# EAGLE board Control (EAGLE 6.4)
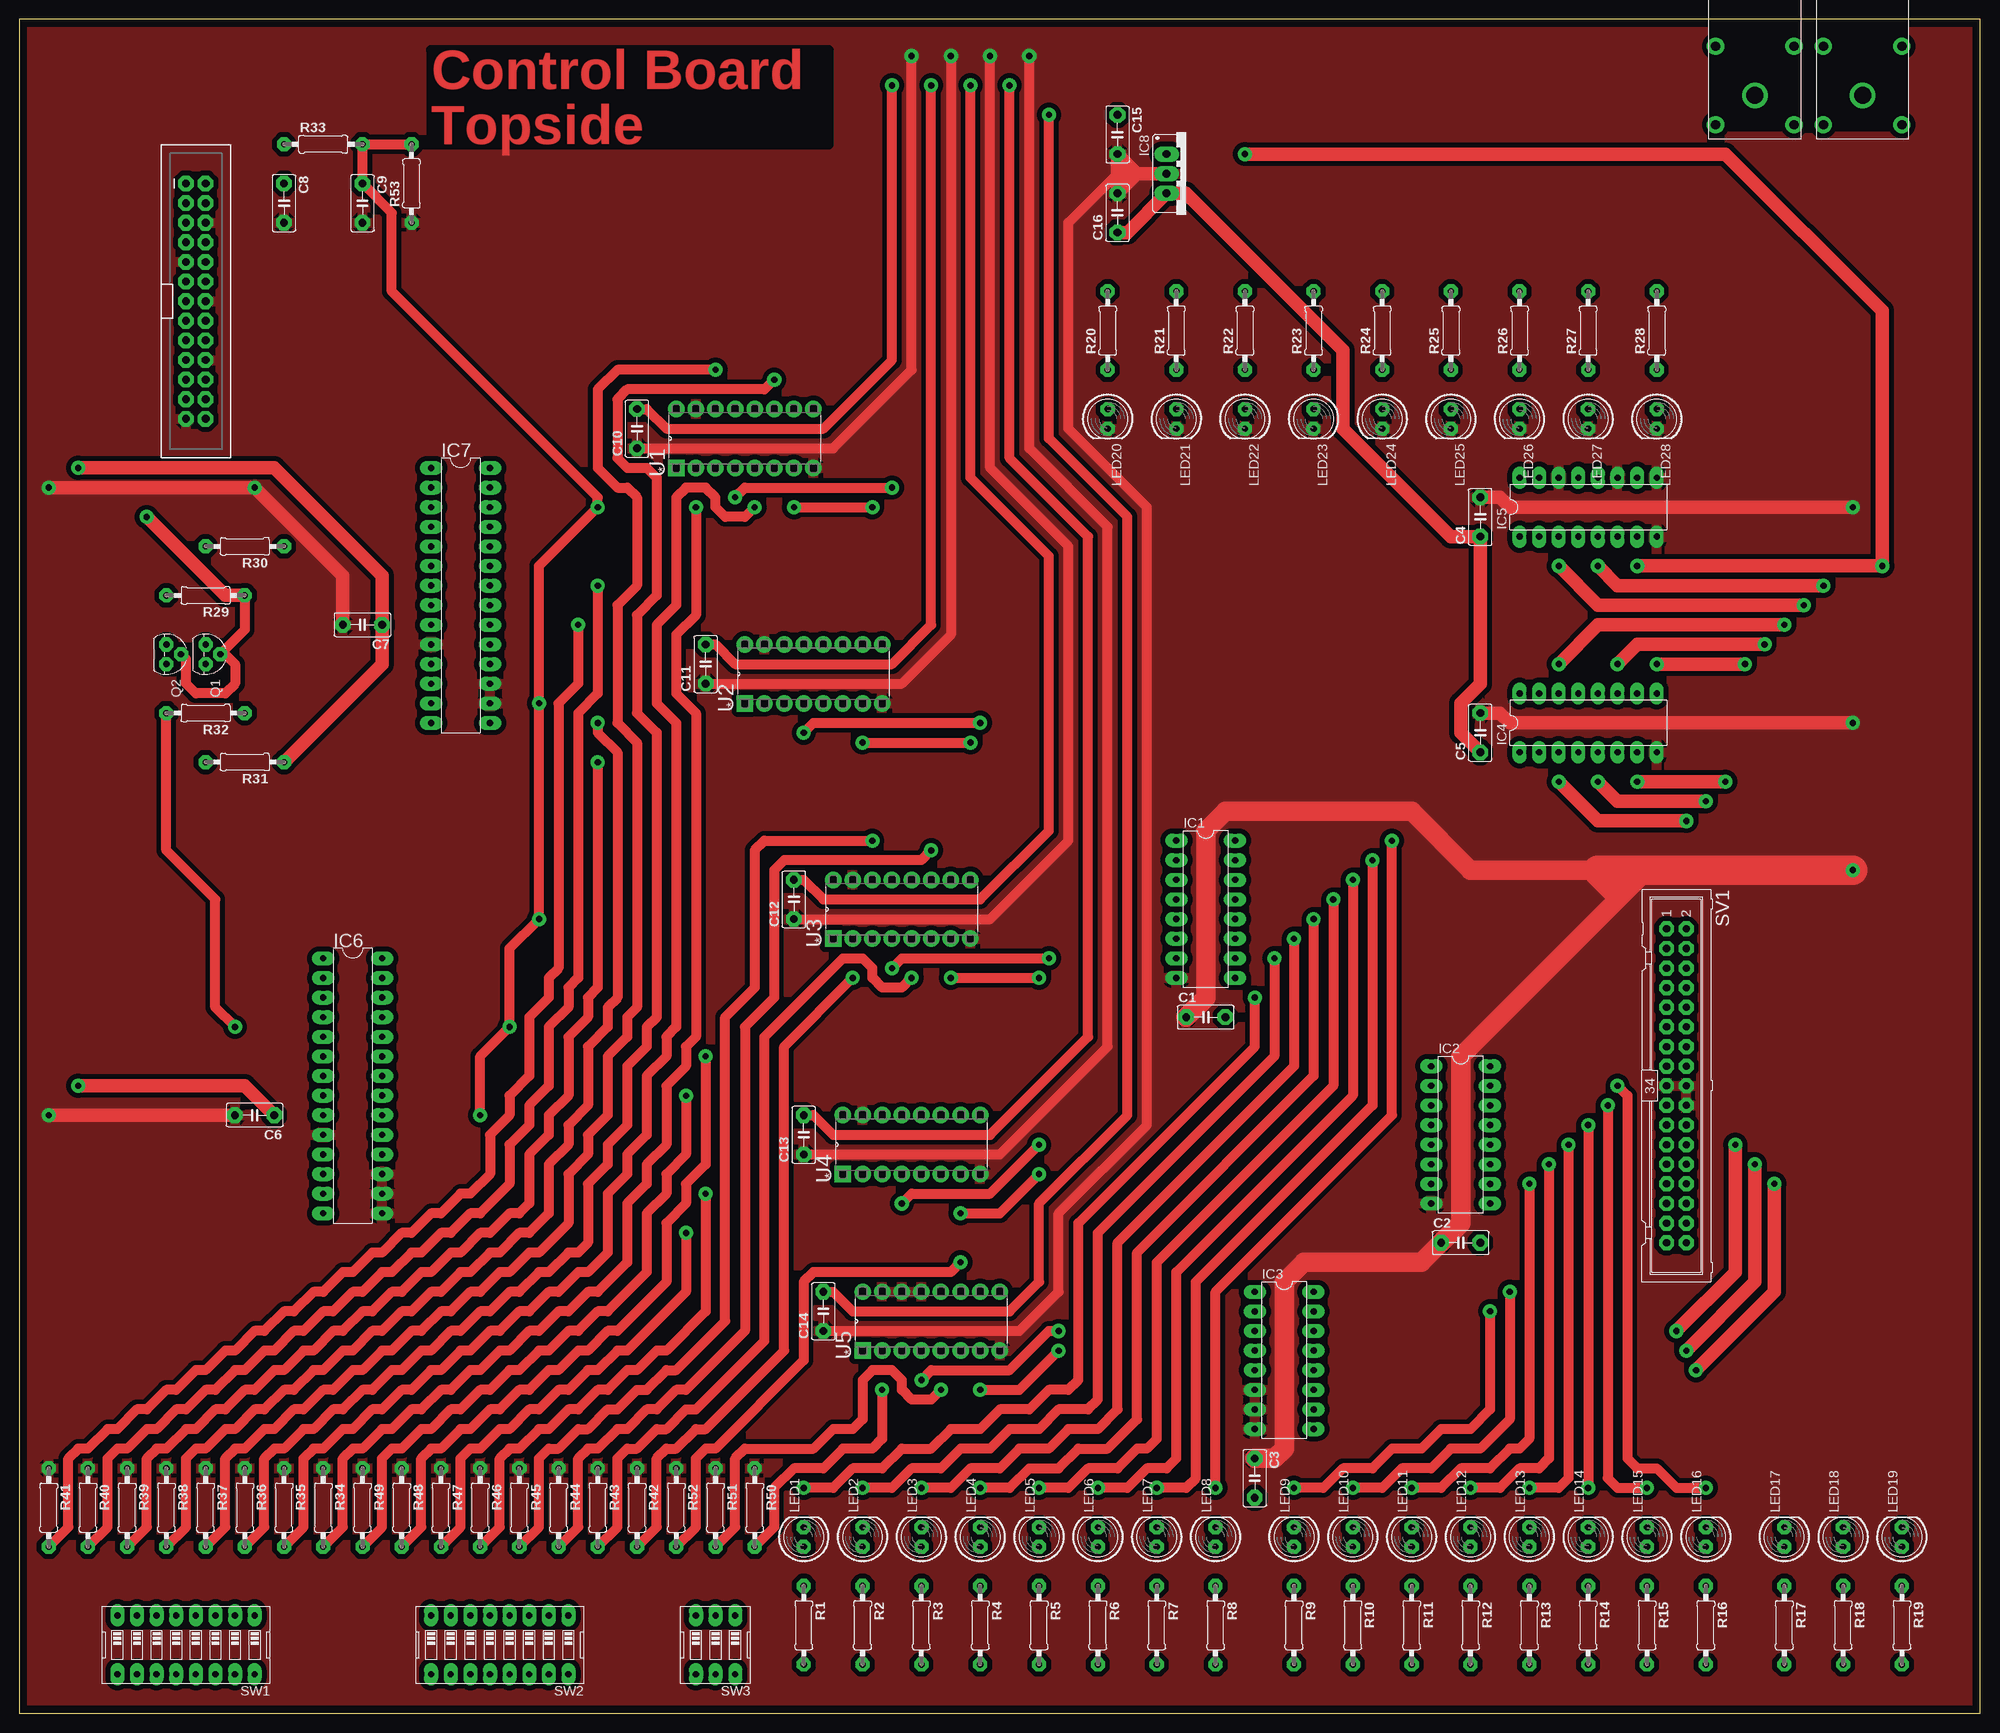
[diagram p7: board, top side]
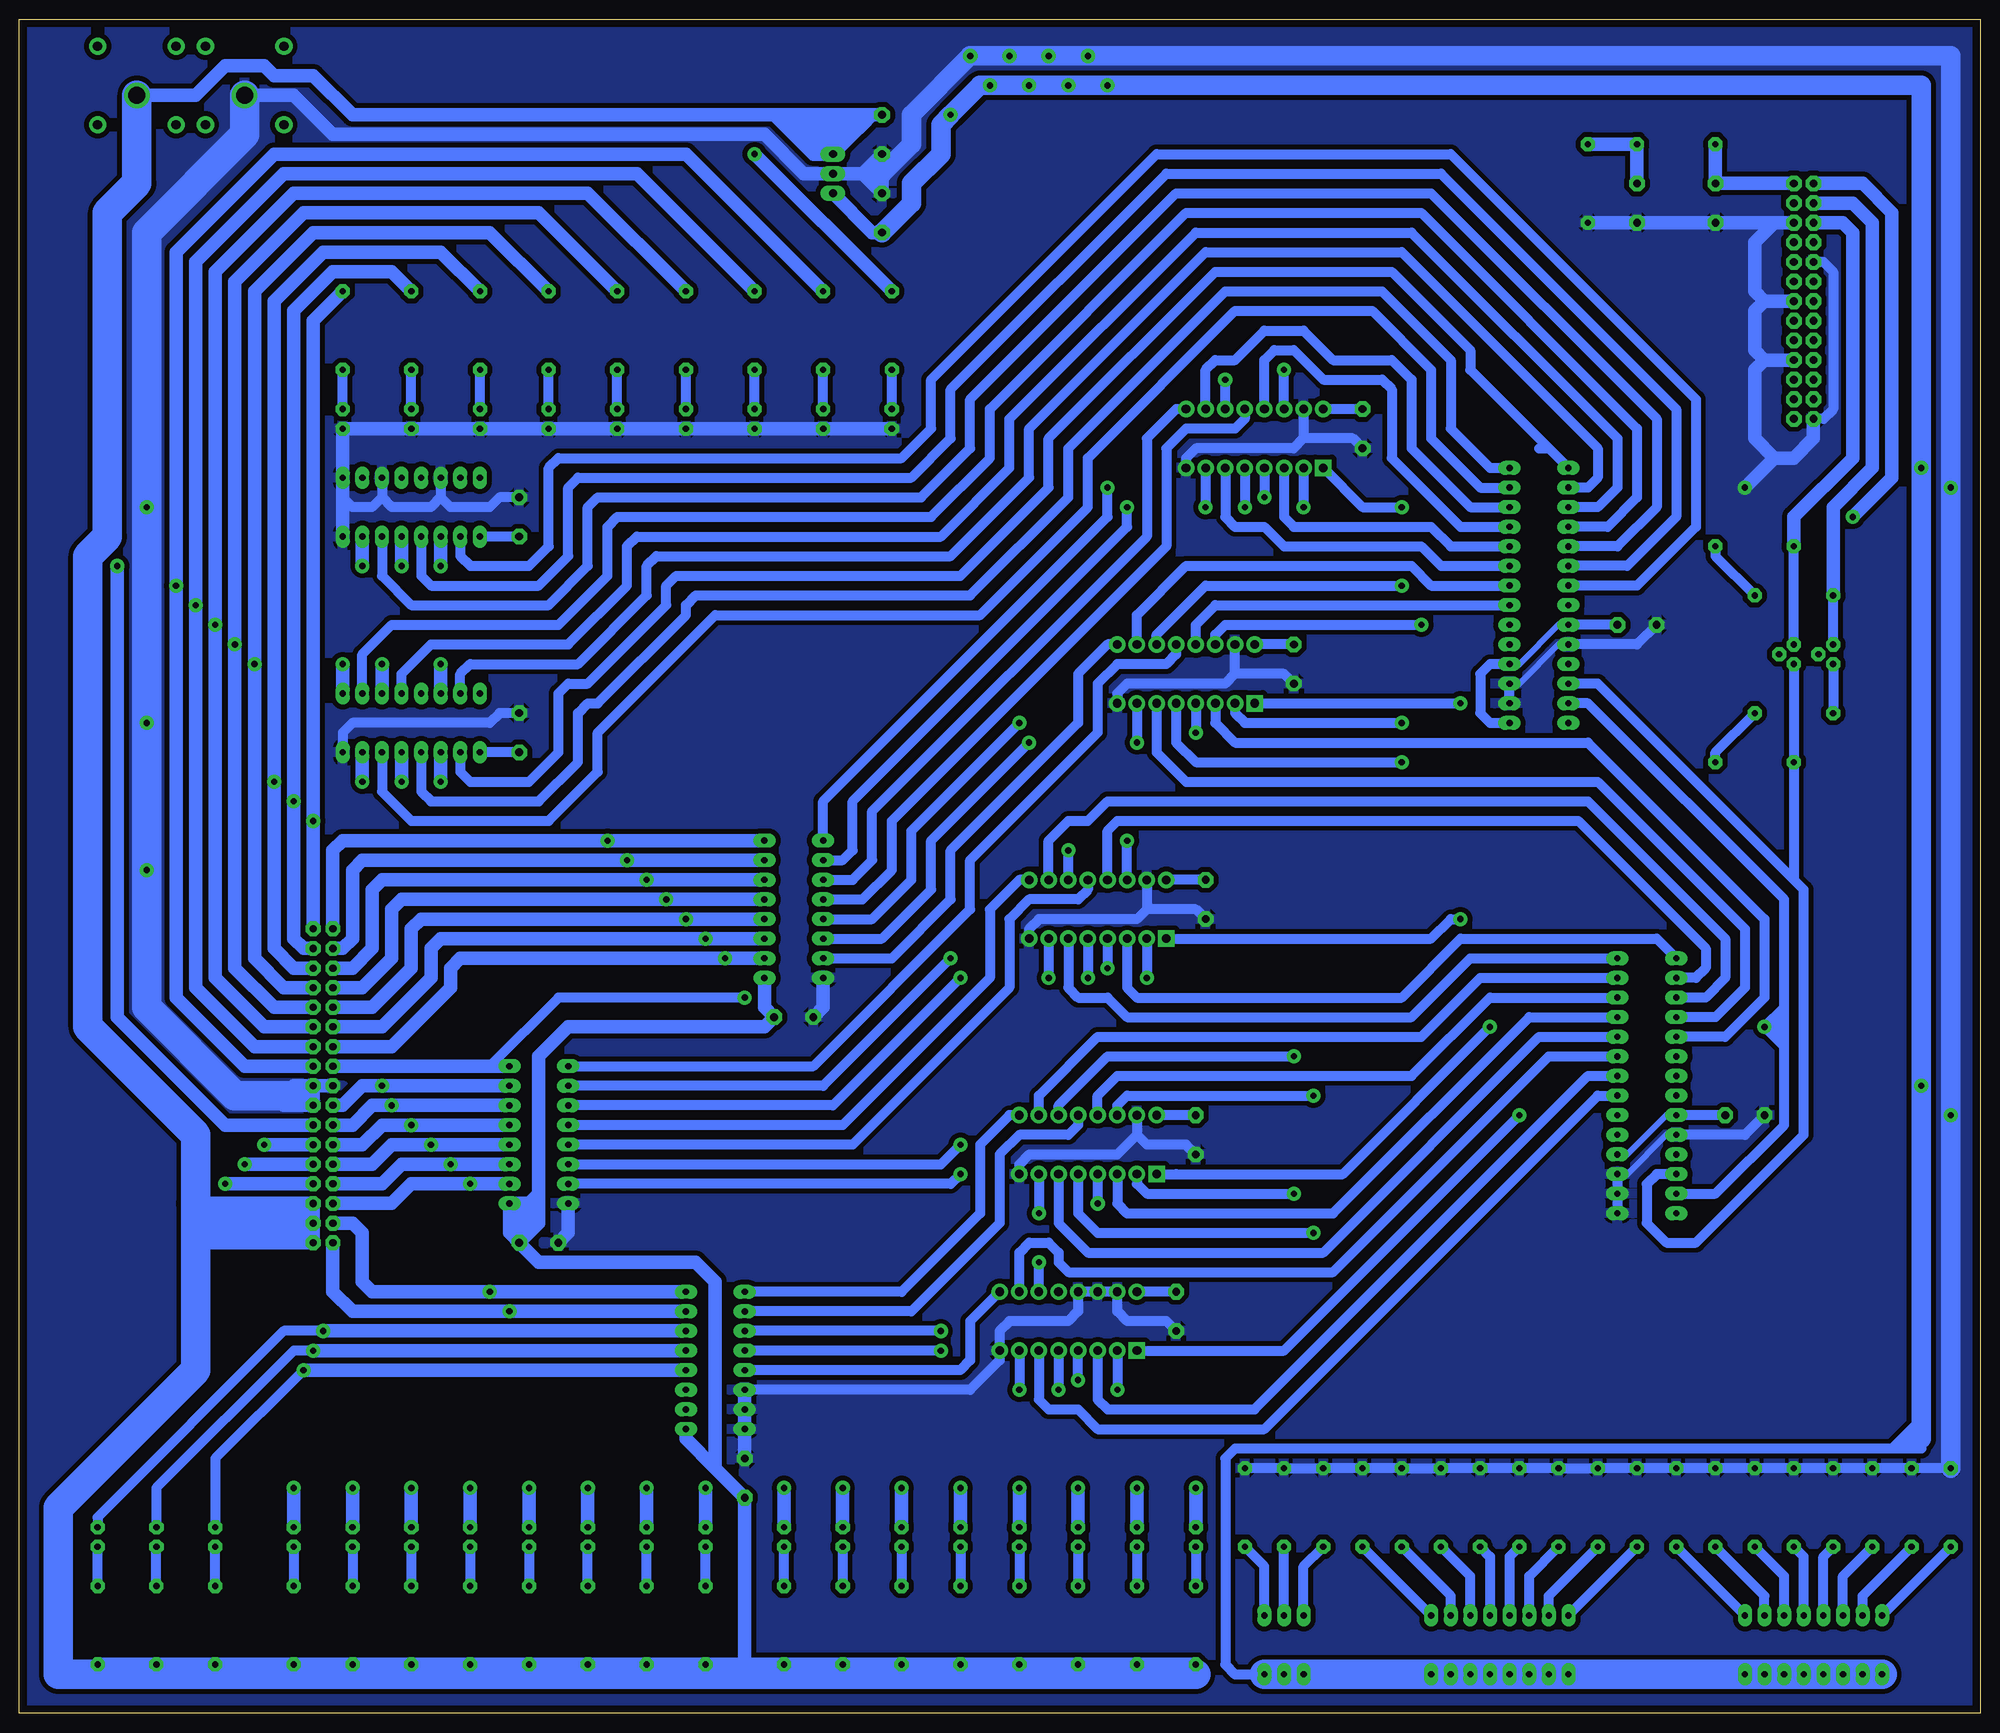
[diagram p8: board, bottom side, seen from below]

Size 253.98 x 219.38 mm. Coordinates in mm from the lower left corner, seen from the top.
Outline: 0,0 253.98,0 253.98,219.38 0,219.38 0,0
Copper layers (1*16): Top 0.035mm / dielectric 1.5mm / Bottom 0.035mm
Design rules "arm-rules-modified": minimum track width 20mil, minimum drill 24mil, track to track 25mil, track to pad 20mil, pad to pad 15mil, via to via 20mil, smd to smd 8mil, copper to edge 40mil, drill to drill 12mil, minimum pad ring 20mil, minimum via ring 20mil, stop-mask expansion 0mil, vias tented up to drill 0mil, thermal gap 15mil
Net classes: 1 12V_Power: width 0.762 mm; 2 Ground: width 0.762 mm; 3 Relay_Interconnects: width 0.762 mm

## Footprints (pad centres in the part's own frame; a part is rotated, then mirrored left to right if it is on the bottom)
C050-030-075 = drill 1 octagon: 1 -2.54,0; 2 2.54,0
DIL16 = drill 0.813 long: 1 -8.89,-3.81; 2 -6.35,-3.81; 3 -3.81,-3.81; 4 -1.27,-3.81; 5 1.27,-3.81; 6 3.81,-3.81; 7 6.35,-3.81; 8 8.89,-3.81; 9 8.89,3.81; 10 6.35,3.81; 11 3.81,3.81; 12 1.27,3.81; 13 -1.27,3.81; 14 -3.81,3.81; 15 -6.35,3.81; 16 -8.89,3.81
DIL28-3 = drill 0.813 long: 1 -16.51,-3.81; 2 -13.97,-3.81; 3 -11.43,-3.81; 4 -8.89,-3.81; 5 -6.35,-3.81; 6 -3.81,-3.81; 7 -1.27,-3.81; 8 1.27,-3.81; 9 3.81,-3.81; 10 6.35,-3.81; 11 8.89,-3.81; 12 11.43,-3.81; 13 13.97,-3.81; 14 16.51,-3.81; 15 16.51,3.81; 16 13.97,3.81; 17 11.43,3.81; 18 8.89,3.81; 19 6.35,3.81; 20 3.81,3.81; 21 1.27,3.81; 22 -1.27,3.81; 23 -3.81,3.81; 24 -6.35,3.81; 25 -8.89,3.81; 26 -11.43,3.81; 27 -13.97,3.81; 28 -16.51,3.81
78XXS = drill 1.016 long: GND 0,-2.54; IN -2.54,-2.54; OUT 2.54,-2.54
2X13-SHROUDED = drill 1.016 pad 1.88 octagon: 1 -1.27,15.24; 2 1.27,15.24; 3 -1.27,12.7; 4 1.27,12.7; 5 -1.27,10.16; 6 1.27,10.16; 7 -1.27,7.62; 8 1.27,7.62; 9 -1.27,5.08; 10 1.27,5.08; 11 -1.27,2.54; 12 1.27,2.54; 13 -1.27,0; 14 1.27,0; 15 -1.27,-2.54; 16 1.27,-2.54; 17 -1.27,-5.08; 18 1.27,-5.08; 19 -1.27,-7.62; 20 1.27,-7.62; 21 -1.27,-10.16; 22 1.27,-10.16; 23 -1.27,-12.7; 24 1.27,-12.7; 25 -1.27,-15.24; 26 1.27,-15.24
LED5MM = drill 0.813 octagon: A -1.27,0; K 1.27,0
TO-92 = drill 0.813 octagon: 1 -1.27,0; 2 0,1.905; 3 1.27,0
0207/10 = drill 0.8 octagon: 1 -5.08,0; 2 5.08,0
ML34 = drill 0.914 octagon: 1 -20.32,-1.27; 2 -20.32,1.27; 3 -17.78,-1.27; 4 -17.78,1.27; 5 -15.24,-1.27; 6 -15.24,1.27; 7 -12.7,-1.27; 8 -12.7,1.27; 9 -10.16,-1.27; 10 -10.16,1.27; 11 -7.62,-1.27; 12 -7.62,1.27; 13 -5.08,-1.27; 14 -5.08,1.27; 15 -2.54,-1.27; 16 -2.54,1.27; 17 0,-1.27; 18 0,1.27; 19 2.54,-1.27; 20 2.54,1.27; 21 5.08,-1.27; 22 5.08,1.27; 23 7.62,-1.27; 24 7.62,1.27; 25 10.16,-1.27; 26 10.16,1.27; 27 12.7,-1.27; 28 12.7,1.27; 29 15.24,-1.27; 30 15.24,1.27; 31 17.78,-1.27; 32 17.78,1.27; 33 20.32,-1.27; 34 20.32,1.27
EDG-08 = drill 0.813 long: 1 -8.89,-3.81; 2 -6.35,-3.81; 3 -3.81,-3.81; 4 -1.27,-3.81; 5 1.27,-3.81; 6 3.81,-3.81; 7 6.35,-3.81; 8 8.89,-3.81; 9 8.89,3.81; 10 6.35,3.81; 11 3.81,3.81; 12 1.27,3.81; 13 -1.27,3.81; 14 -3.81,3.81; 15 -6.35,3.81; 16 -8.89,3.81
EDG-03 = drill 0.813 long: 1 -2.54,-3.81; 2 0,-3.81; 3 2.54,-3.81; 4 2.54,3.81; 5 0,3.81; 6 -2.54,3.81
DIP254P762X508-16 = drill 1.118 square: 1 -7.62,17.78 | drill 1.118: 2 -7.62,15.24; 3 -7.62,12.7; 4 -7.62,10.16; 5 -7.62,7.62; 6 -7.62,5.08; 7 -7.62,2.54; 8 -7.62,0; 9 0,0; 10 0,2.54; 11 0,5.08; 12 0,7.62; 13 0,10.16; 14 0,12.7; 15 0,15.24; 16 0,17.78
BANPLUG = drill 2.2: 1 0,-6.36 | drill 1.2: P$1 -5.08,-10.16; P$2 5.08,-10.16; P$3 -5.08,0; P$4 5.08,0

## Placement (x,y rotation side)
C1  [C050-030-075]  153.67,90.17 0 top
C2  [C050-030-075]  186.69,60.96 0 top
C3  [C050-030-075]  160.02,30.48 270 top
C4  [C050-030-075]  189.23,154.94 90 top
C5  [C050-030-075]  189.23,127 90 top
C6  [C050-030-075]  30.48,77.47 180 top
C7  [C050-030-075]  44.45,140.97 180 top
C8  22n  [C050-030-075]  34.29,195.58 270 top
C9  22n  [C050-030-075]  44.45,195.58 270 top
C10  [C050-030-075]  80.01,166.37 90 top
C11  [C050-030-075]  88.9,135.89 90 top
C12  [C050-030-075]  100.33,105.41 90 top
C13  [C050-030-075]  101.6,74.93 90 top
C14  [C050-030-075]  104.14,52.07 90 top
C15  [C050-030-075]  142.24,204.47 270 top
C16  [C050-030-075]  142.24,194.31 90 top
IC1  ULN2003AN  [DIL16]  153.67,104.14 270 top
IC2  ULN2003AN  [DIL16]  186.69,74.93 270 top
IC3  ULN2003AN  [DIL16]  163.83,45.72 270 top
IC4  4049N  [DIL16]  203.2,128.27 0 top
IC5  4049N  [DIL16]  203.2,156.21 0 top
IC6  MCP23017SP  [DIL28-3]  43.18,81.28 270 top
IC7  MCP23017SP  [DIL28-3]  57.15,144.78 270 top
IC8  [78XXS]  151.13,199.39 270 top
JP1  RASPBERRYPI-GPIOPTH  [2X13-SHROUDED]  22.86,182.88 0 top
LED1  [LED5MM]  101.6,22.86 90 top
LED2  [LED5MM]  109.22,22.86 90 top
LED3  [LED5MM]  116.84,22.86 90 top
LED4  [LED5MM]  124.46,22.86 90 top
LED5  [LED5MM]  132.08,22.86 90 top
LED6  [LED5MM]  139.7,22.86 90 top
LED7  [LED5MM]  147.32,22.86 90 top
LED8  [LED5MM]  154.94,22.86 90 top
LED9  [LED5MM]  165.1,22.86 90 top
LED10  [LED5MM]  172.72,22.86 90 top
LED11  [LED5MM]  180.34,22.86 90 top
LED12  [LED5MM]  187.96,22.86 90 top
LED13  [LED5MM]  195.58,22.86 90 top
LED14  [LED5MM]  203.2,22.86 90 top
LED15  [LED5MM]  210.82,22.86 90 top
LED16  [LED5MM]  218.44,22.86 90 top
LED17  [LED5MM]  228.6,22.86 90 top
LED18  [LED5MM]  236.22,22.86 90 top
LED19  [LED5MM]  243.84,22.86 90 top
LED20  [LED5MM]  140.97,167.64 270 top
LED21  [LED5MM]  149.86,167.64 270 top
LED22  [LED5MM]  158.75,167.64 270 top
LED23  [LED5MM]  167.64,167.64 270 top
LED24  [LED5MM]  176.53,167.64 270 top
LED25  [LED5MM]  185.42,167.64 270 top
LED26  [LED5MM]  194.31,167.64 270 top
LED27  [LED5MM]  203.2,167.64 270 top
LED28  [LED5MM]  212.09,167.64 270 top
Q1  TN0602N3  [TO-92]  24.13,137.16 270 top
Q2  TN0602N3  [TO-92]  19.05,137.16 270 top
R1  510  [0207/10]  101.6,11.43 270 top
R2  510  [0207/10]  109.22,11.43 270 top
R3  510  [0207/10]  116.84,11.43 270 top
R4  510  [0207/10]  124.46,11.43 270 top
R5  510  [0207/10]  132.08,11.43 270 top
R6  510  [0207/10]  139.7,11.43 270 top
R7  510  [0207/10]  147.32,11.43 270 top
R8  510  [0207/10]  154.94,11.43 270 top
R9  510  [0207/10]  165.1,11.43 270 top
R10  510  [0207/10]  172.72,11.43 270 top
R11  510  [0207/10]  180.34,11.43 270 top
R12  510  [0207/10]  187.96,11.43 270 top
R13  510  [0207/10]  195.58,11.43 270 top
R14  510  [0207/10]  203.2,11.43 270 top
R15  510  [0207/10]  210.82,11.43 270 top
R16  510  [0207/10]  218.44,11.43 270 top
R17  510  [0207/10]  228.6,11.43 270 top
R18  510  [0207/10]  236.22,11.43 270 top
R19  510  [0207/10]  243.84,11.43 270 top
R20  510  [0207/10]  140.97,179.07 90 top
R21  510  [0207/10]  149.86,179.07 90 top
R22  510  [0207/10]  158.75,179.07 90 top
R23  510  [0207/10]  167.64,179.07 90 top
R24  510  [0207/10]  176.53,179.07 90 top
R25  510  [0207/10]  185.42,179.07 90 top
R26  510  [0207/10]  194.31,179.07 90 top
R27  510  [0207/10]  203.2,179.07 90 top
R28  510  [0207/10]  212.09,179.07 90 top
R29  10k  [0207/10]  24.13,144.78 180 top
R30  10k  [0207/10]  29.21,151.13 180 top
R31  10k  [0207/10]  29.21,123.19 180 top
R32  10k  [0207/10]  24.13,129.54 180 top
R33  100  [0207/10]  39.37,203.2 0 top
R34  10k  [0207/10]  39.37,26.67 270 top
R35  10k  [0207/10]  34.29,26.67 270 top
R36  10k  [0207/10]  29.21,26.67 270 top
R37  10k  [0207/10]  24.13,26.67 270 top
R38  10k  [0207/10]  19.05,26.67 270 top
R39  10k  [0207/10]  13.97,26.67 270 top
R40  10k  [0207/10]  8.89,26.67 270 top
R41  10k  [0207/10]  3.81,26.67 270 top
R42  10k  [0207/10]  80.01,26.67 270 top
R43  10k  [0207/10]  74.93,26.67 270 top
R44  10k  [0207/10]  69.85,26.67 270 top
R45  10k  [0207/10]  64.77,26.67 270 top
R46  10k  [0207/10]  59.69,26.67 270 top
R47  10k  [0207/10]  54.61,26.67 270 top
R48  10k  [0207/10]  49.53,26.67 270 top
R49  10k  [0207/10]  44.45,26.67 270 top
R50  10k  [0207/10]  95.25,26.67 270 top
R51  10k  [0207/10]  90.17,26.67 270 top
R52  10k  [0207/10]  85.09,26.67 270 top
R53  10k  [0207/10]  50.8,198.12 90 top
SV1  [ML34]  214.63,81.28 270 top
SW1  [EDG-08]  21.59,8.89 180 top
SW2  [EDG-08]  62.23,8.89 180 top
SW3  [EDG-03]  90.17,8.89 180 top
U1  SN74AHC157N  [DIP254P762X508-16]  102.87,168.91 90 top
U2  SN74AHC157N  [DIP254P762X508-16]  111.76,138.43 90 top
U3  SN74AHC157N  [DIP254P762X508-16]  123.19,107.95 90 top
U4  SN74AHC157N  [DIP254P762X508-16]  124.46,77.47 90 top
U5  SN74AHC157N  [DIP254P762X508-16]  127,54.61 90 top
U$1  BANANACONNECTOR  [BANPLUG]  238.76,215.9 0 top
U$2  BANANACONNECTOR  [BANPLUG]  224.79,215.9 0 top

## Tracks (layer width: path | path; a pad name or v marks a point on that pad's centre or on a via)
+3V3  (via drill 0.8)
  Top 1.27: Q2.2 21.59,136.53 21.59,133.35 22.86,132.08 26.67,132.08 27.94,133.35 27.94,135.89 26.67,137.16 Q1.2 29.21,140.34 R29.1
  Top 1.778: v16.51,154.94 26.67,144.78 R29.1
  Bottom 1.27: R30.1 34.29,149.86 R29.1
  Bottom 1.778: JP1.1 15.24,198.12 11.43,194.31 11.43,160.02 v16.51,154.94
+5V  (via drill 0.8)
  Top 1.27: C10.2 81.28,168.91 83.82,166.37 104.14,166.37 113.03,175.26 v113.03,210.82 | C11.2 90.17,138.43 92.71,135.89 113.03,135.89 118.11,140.97 v118.11,210.82 | C13.2 102.87,77.47 105.41,74.93 125.73,74.93 138.43,87.63 138.43,152.4 128.27,162.56 v128.27,210.82 | C14.2 105.41,54.61 107.95,52.07 128.27,52.07 132.08,55.88 132.08,66.04 143.51,77.47 143.51,154.94 133.35,165.1 v133.35,207.01 | C12.2 101.6,107.95 104.14,105.41 124.46,105.41 133.35,114.3 133.35,149.86 123.19,160.02 v123.19,210.82
  Top 1.778: C5.1 186.69,127 186.69,130.81 189.23,133.35 C4.1 185.42,152.4 171.45,166.37 171.45,176.53 151.13,196.85 IC8.OUT 143.51,191.77 C16.1 | C6.1 29.21,81.28 v7.62,81.28 | v7.62,161.29 33.02,161.29 46.99,147.32 C7.1 46.99,135.89 R31.1
  Bottom 0.813: IC6.9 40.64,77.47 45.72,72.39 IC6.18 | IC7.9 54.61,140.97 59.69,135.89 IC7.18
  Bottom 1.27: R31.1 34.29,124.46 R32.1 | C6.1 IC6.9 | C7.1 IC7.9 | IC7.18 63.5,135.89 64.77,134.62 64.77,129.54 63.5,128.27 IC7.15 | C10.2 U1.16 | C11.2 U2.16 | C12.2 U3.16 | C13.2 U4.16 | C14.2 U5.16 | C5.1 IC4.1 | C4.1 IC5.1 | 10.16,34.29 7.62,34.29 7.62,35.56 8.89,35.56 10.16,34.29 | 10.16,34.29 11.43,34.29 | 11.43,34.29 96.52,34.29 97.79,33.02 97.79,6.35 96.52,5.08 SW3.6 | 7.62,38.1 11.43,34.29
  Bottom 1.778: C16.1 143.51,191.77 IC8.OUT | SW2.16 SW3.4
  Bottom 2.54: SW2.16 SW2.15 | 54.61,5.08 SW2.9 | C16.1 138.43,195.58 138.43,198.12 134.62,201.93 134.62,205.74 v133.35,207.01 129.54,210.82 v128.27,210.82 v123.19,210.82 v118.11,210.82 v113.03,210.82 7.62,210.82 v7.62,161.29 v7.62,81.28 7.62,38.1 7.62,35.56
  Bottom 3.81: SW3.6 SW3.5 SW3.4 SW2.15 SW2.14 SW2.13 SW2.12 SW2.11 SW2.10 54.61,5.08 SW1.16 SW1.15 SW1.14 SW1.13 SW1.12 SW1.11 SW1.10 SW1.9
+12V
  Bottom 1.27: R5.2 R6.2 139.7,5.08
  Bottom 1.778: R19.2 R18.2 R17.2 R16.2 R15.2 R14.2 R13.2 R12.2 R11.2 R10.2 R9.2 160.02,6.35 | R1.2 R2.2 R3.2 R4.2 R5.2 R7.2 R8.2 160.02,6.35 | IC1.9 157.48,91.44 C1.2 157.48,88.9 182.88,88.9 186.69,85.09 186.69,67.31 | C2.2 190.5,62.23 190.5,64.77 | 190.5,64.77 IC2.9 187.96,66.04 186.69,67.31 | 160.02,6.35 C3.2 163.83,31.75 | 163.83,31.75 167.64,35.56 IC3.9 | 163.83,31.75 163.83,55.88 166.37,58.42 186.69,58.42 C2.2 | 186.69,67.31 186.69,64.77 | 186.69,64.77 186.69,63.5 C2.2 | C2.2 189.23,62.23 186.69,64.77 | 186.69,64.77 190.5,64.77 | 190.5,64.77 189.23,63.5 | U$1.1 231.14,209.55 227.33,213.36 222.25,213.36 220.98,212.09 215.9,212.09 210.82,207.01 156.21,207.01 | 144.78,205.74 143.51,207.01 C15.1 156.21,207.01 | 144.78,205.74 146.05,204.47 | 146.05,204.47 147.32,203.2 | 147.32,203.2 IC8.IN 151.13,201.93 152.4,203.2 | 156.21,207.01 154.94,205.74 | 154.94,205.74 153.67,204.47 | 153.67,204.47 152.4,203.2 | 144.78,205.74 154.94,205.74 | 146.05,204.47 153.67,204.47 | 147.32,203.2 152.4,203.2 | SV1.32 SV1.30 231.14,66.04 | SV1.32 SV1.34 229.87,60.96 | 217.17,63.5 SV1.32
  Bottom 3.81: 231.14,66.04 231.14,74.93 245.11,88.9 245.11,149.86 242.57,152.4 242.57,194.31 238.76,198.12 U$1.1 | 231.14,66.04 231.14,44.45 248.92,26.67 248.92,5.08 139.7,5.08 101.6,5.08 | 231.14,66.04 228.6,63.5 217.17,63.5
A_0  (via drill 0.8)
  Top 1.27: v92.71,157.48 93.98,158.75 v113.03,158.75
  Bottom 1.27: U1.4 v92.71,157.48 | IC1.1 149.86,118.11 113.03,154.94 v113.03,158.75
A_1  (via drill 0.8)
  Top 1.27: v100.33,156.21 v110.49,156.21
  Bottom 1.27: U1.7 v100.33,156.21 | IC1.2 147.32,110.49 146.05,111.76 146.05,118.11 110.49,153.67 v110.49,156.21
A_2
  Bottom 1.27: U1.9 104.14,168.91 107.95,165.1 107.95,152.4 143.51,116.84 143.51,110.49 146.05,107.95 IC1.3
A_3
  Bottom 1.27: U1.12 95.25,167.64 96.52,166.37 102.87,166.37 105.41,163.83 105.41,151.13 140.97,115.57 140.97,109.22 144.78,105.41 IC1.4
A_4  (via drill 0.8)
  Top 1.27: v101.6,127 102.87,128.27 v124.46,128.27
  Bottom 1.27: U2.4 v101.6,127 | IC1.5 143.51,102.87 138.43,107.95 138.43,114.3 v124.46,128.27
A_5  (via drill 0.8)
  Top 1.27: v109.22,125.73 v123.19,125.73
  Bottom 1.27: U2.7 v109.22,125.73 | IC1.6 142.24,100.33 135.89,106.68 135.89,113.03 v123.19,125.73
A_6
  Bottom 1.27: U2.9 113.03,138.43 116.84,134.62 116.84,128.27 133.35,111.76 133.35,105.41 140.97,97.79 IC1.7
A_7
  Bottom 1.27: U2.12 104.14,137.16 105.41,135.89 111.76,135.89 114.3,133.35 114.3,127 130.81,110.49 130.81,104.14 151.13,83.82 IC2.1
B_0  (via drill 0.8)
  Top 1.27: v113.03,96.52 114.3,97.79 v133.35,97.79
  Bottom 1.27: U3.4 v113.03,96.52 | v133.35,97.79 149.86,81.28 IC2.2
B_1  (via drill 0.8)
  Top 1.27: v120.65,95.25 v132.08,95.25
  Bottom 1.27: U3.7 v120.65,95.25 | v132.08,95.25 148.59,78.74 IC2.3
B_2
  Bottom 1.27: U3.9 124.46,107.95 128.27,104.14 128.27,95.25 147.32,76.2 IC2.4
B_3
  Bottom 1.27: U3.12 115.57,106.68 116.84,105.41 123.19,105.41 125.73,102.87 125.73,93.98 146.05,73.66 IC2.5
B_4  (via drill 0.8)
  Top 1.27: v114.3,66.04 115.57,67.31 125.73,67.31 v132.08,73.66
  Bottom 1.27: U4.4 v114.3,66.04 | IC2.6 134.62,71.12 v132.08,73.66
B_5  (via drill 0.8)
  Top 1.27: v121.92,64.77 127,64.77 v132.08,69.85
  Bottom 1.27: U4.7 v121.92,64.77 | v132.08,69.85 133.35,68.58 IC2.7
B_6
  Bottom 1.27: U4.9 125.73,77.47 129.54,73.66 129.54,64.77 139.7,54.61 IC3.1
B_7
  Bottom 1.27: U4.12 116.84,76.2 118.11,74.93 124.46,74.93 127,72.39 127,63.5 138.43,52.07 IC3.2
CARRY_OUT  (via drill 0.8)
  Top 1.778: v209.55,148.59 v241.3,148.59 241.3,181.61 220.98,201.93 v158.75,201.93
  Bottom 1.778: SV1.22 227.33,76.2 241.3,90.17 v241.3,148.59 | R20.2 v158.75,201.93 | IC5.7 v209.55,148.59
GND  (via drill 0.8)
  Top 1.27: C10.1 105.41,163.83 115.57,173.99 v115.57,214.63 | C11.1 114.3,133.35 120.65,139.7 v120.65,214.63 | C13.1 127,72.39 140.97,86.36 140.97,153.67 130.81,163.83 v130.81,214.63 | C14.1 129.54,49.53 134.62,54.61 134.62,64.77 146.05,76.2 146.05,156.21 135.89,166.37 135.89,193.04 142.24,199.39 | C12.1 125.73,102.87 135.89,113.03 135.89,151.13 125.73,161.29 v125.73,214.63
  Top 1.778: v237.49,156.21 193.04,156.21 191.77,157.48 C4.2 | C5.2 191.77,129.54 193.04,128.27 v237.49,128.27 | 142.24,199.39 C15.2 144.78,199.39 | 142.24,199.39 C16.2 144.78,199.39 | 142.24,199.39 144.78,199.39 | 144.78,199.39 IC8.GND | C6.2 v3.81,77.47 | C7.2 41.91,147.32 v30.48,158.75 v3.81,158.75
  Top 2.54: C1.1 153.67,92.71 153.67,114.3 156.21,116.84 180.34,116.84 187.96,109.22 204.47,109.22 | C3.1 162.56,33.02 163.83,34.29 163.83,55.88 166.37,58.42 181.61,58.42 C2.1 186.69,63.5 186.69,85.09 210.82,109.22
  Top 3.81: v237.49,109.22 210.82,109.22 204.47,109.22 207.01,106.68
  Bottom 0.813: IC6.10 40.64,74.93 45.72,69.85 IC6.17 | IC7.10 54.61,138.43 59.69,133.35 IC7.17
  Bottom 1.27: R50.1 R51.1 R52.1 R42.1 R43.1 R44.1 R45.1 R46.1 R47.1 R48.1 R49.1 R34.1 R35.1 R36.1 R37.1 R38.1 R39.1 R40.1 R41.1 | C6.2 30.48,74.93 IC6.10 | IC6.17 IC6.16 IC6.15 | C7.2 44.45,138.43 IC7.10 | IC7.16 IC7.17 | C10.1 81.28,165.1 87.63,165.1 | U1.15 87.63,165.1 | 87.63,165.1 88.9,163.83 101.6,163.83 102.87,162.56 U1.8 | C11.1 90.17,134.62 96.52,134.62 | 96.52,134.62 U2.15 | 96.52,134.62 97.79,133.35 110.49,133.35 111.76,132.08 U2.8 | C12.1 101.6,104.14 107.95,104.14 | U3.15 107.95,104.14 | 107.95,104.14 109.22,102.87 121.92,102.87 123.19,101.6 U3.8 | C13.1 102.87,73.66 107.95,73.66 109.22,74.93 | U4.15 109.22,74.93 | C14.1 105.41,50.8 110.49,50.8 111.76,52.07 U5.15 U5.14 U5.13 116.84,52.07 118.11,50.8 125.73,50.8 127,49.53 U5.8 127,45.72 130.81,41.91 IC3.6 | C5.2 191.77,129.54 193.04,128.27 210.82,128.27 212.09,127 IC4.8 | C4.2 191.77,157.48 193.04,156.21 198.12,156.21 199.39,157.48 | IC5.14 199.39,157.48 | 199.39,157.48 200.66,156.21 205.74,156.21 207.01,157.48 | IC5.11 207.01,157.48 | 207.01,157.48 208.28,156.21 210.82,156.21 212.09,157.48 IC5.9 | U4.8 124.46,71.12 123.19,72.39 111.76,72.39 109.22,74.93 | JP1.9 20.32,187.96 19.05,186.69 19.05,168.91 20.32,167.64 JP1.25
  Bottom 1.778: LED20.K LED21.K LED22.K LED23.K LED24.K LED25.K LED26.K LED27.K LED28.K IC5.9 IC5.8 | 144.78,199.39 C15.2 142.24,199.39 C16.2 | C16.2 144.78,199.39 | C16.2 143.51,198.12 143.51,199.39 144.78,199.39 | R53.1 C9.2 C8.2 26.67,193.04 | IC1.8 149.86,91.44 C1.1 | C2.1 182.88,62.23 IC2.8 | IC3.6 IC3.7 IC3.8 C3.1 | U$2.1 218.44,209.55 213.36,204.47 157.48,204.47 152.4,199.39 IC8.GND 144.78,199.39 | JP1.25 21.59,165.1 24.13,162.56 26.67,162.56 | 26.67,162.56 v30.48,158.75 | JP1.6 26.67,193.04 | 26.67,193.04 29.21,190.5 29.21,184.15 27.94,182.88 | 27.94,182.88 JP1.14 | 27.94,182.88 29.21,181.61 29.21,176.53 27.94,175.26 | 27.94,175.26 JP1.20 | 27.94,175.26 29.21,173.99 29.21,165.1 26.67,162.56 | SV1.17 SV1.18 | SV1.18 SV1.20 219.71,78.74 | 217.17,80.01 215.9,80.01 SV1.18 | SV1.18 218.44,81.28
  Bottom 2.54: 142.24,199.39 138.43,203.2 138.43,207.01 v130.81,214.63 v125.73,214.63 v120.65,214.63 v115.57,214.63 3.81,214.63 v3.81,158.75 v3.81,77.47 R41.1
  Bottom 3.81: U$2.1 224.79,204.47 237.49,191.77 v237.49,156.21 v237.49,128.27 v237.49,109.22 237.49,91.44 226.06,80.01 217.17,80.01
  pour Bottom: 0,219.71 254,219.71 254,0 0,0
  pour Top: 0,219.71 254,219.71 254,0 0,0
I_0  (via drill 0.8)
  Top 1.27: v116.84,43.18 118.11,44.45 128.27,44.45 133.35,49.53 v134.62,49.53
  Bottom 1.27: v116.84,43.18 U5.4 | v134.62,49.53 IC3.3
I_1  (via drill 0.8)
  Top 1.27: v124.46,41.91 129.54,41.91 v134.62,46.99
  Bottom 1.27: U5.7 v124.46,41.91 | v134.62,46.99 IC3.4
I_2
  Bottom 1.27: U5.9 130.81,50.8 130.81,45.72 132.08,44.45 IC3.5
N$2
  Bottom 1.27: LED1.A R1.1
N$75
  Bottom 1.27: LED2.A R2.1
N$77
  Bottom 1.27: LED3.A R3.1
N$78
  Bottom 1.27: LED4.A R4.1
N$79
  Bottom 1.27: LED5.A R5.1
N$80
  Bottom 1.27: LED6.A R6.1
N$81
  Bottom 1.27: LED7.A R7.1
N$82
  Bottom 1.27: R8.1 LED8.A
N$83
  Bottom 1.27: Q1.3 R31.2 24.13,107.95 | IC6.12 41.91,69.85 43.18,68.58 43.18,63.5 40.64,60.96 36.83,60.96 22.86,74.93 22.86,106.68 24.13,107.95 | 24.13,107.95 49.53,133.35 IC7.12
N$84
  Bottom 1.27: Q1.1 R30.2
  Bottom 1.778: JP1.5 17.78,193.04 16.51,191.77 16.51,162.56 24.13,154.94 R30.2
N$85  (via drill 0.8)
  Top 1.27: v27.94,88.9 25.4,91.44 25.4,105.41 19.05,111.76 R32.2
  Bottom 1.27: Q2.3 R32.2 | IC6.13 34.29,67.31 25.4,76.2 25.4,86.36 | 25.4,86.36 25.4,87.63 | 25.4,87.63 25.4,88.9 | 25.4,88.9 25.4,90.17 | 25.4,90.17 25.4,91.44 | 25.4,91.44 25.4,105.41 50.8,130.81 IC7.13 | 25.4,88.9 26.67,88.9 | 26.67,88.9 v27.94,88.9 | v27.94,88.9 25.4,86.36 | 25.4,87.63 26.67,88.9 | v27.94,88.9 25.4,91.44 | 25.4,90.17 26.67,88.9
N$86
  Bottom 1.27: Q2.1 R29.2
  Bottom 1.778: R29.2 19.05,156.21 13.97,161.29 13.97,193.04 16.51,195.58 JP1.3
N$91
  Bottom 1.27: R9.1 LED9.A
N$92
  Bottom 1.27: R10.1 LED10.A
N$93
  Bottom 1.27: R11.1 LED11.A
N$94
  Bottom 1.27: LED12.A R12.1
N$95
  Bottom 1.27: LED13.A R13.1
N$96
  Bottom 1.27: LED14.A R14.1
N$97
  Bottom 1.27: LED15.A R15.1
N$98
  Bottom 1.27: LED16.A R16.1
N$107
  Bottom 1.27: R17.1 LED17.A
N$108
  Bottom 1.27: R18.1 LED18.A
N$109
  Bottom 1.27: R19.1 LED19.A
N$113
  Bottom 1.27: LED20.A R20.1
N$114
  Bottom 1.27: LED21.A R21.1
N$115
  Bottom 1.27: LED22.A R22.1
N$116
  Bottom 1.27: LED23.A R23.1
N$117
  Bottom 1.27: LED24.A R24.1
N$118
  Bottom 1.27: LED25.A R25.1
N$119
  Bottom 1.27: LED26.A R26.1
N$120
  Bottom 1.27: LED27.A R27.1
N$122
  Bottom 1.778: R33.1 C8.1 JP1.2
N$129
  Bottom 1.27: LED28.A R28.1
NOT_A_0  (via drill 0.8)
  Top 1.27: v177.8,113.03 177.8,77.47 154.94,54.61 v154.94,29.21
  Bottom 1.778: SV1.1 213.36,111.76 212.09,113.03 v177.8,113.03 IC1.16 | LED8.K v154.94,29.21
NOT_A_1  (via drill 0.8)
  Top 1.27: v175.26,110.49 175.26,78.74 152.4,55.88 152.4,30.48 151.13,29.21 v147.32,29.21
  Bottom 1.778: SV1.3 212.09,99.06 210.82,100.33 210.82,109.22 209.55,110.49 v175.26,110.49 IC1.15 | v147.32,29.21 LED7.K
NOT_A_2  (via drill 0.8)
  Top 1.27: v172.72,107.95 172.72,80.01 149.86,57.15 149.86,33.02 148.59,31.75 146.05,31.75 143.51,29.21 v139.7,29.21
  Bottom 1.778: SV1.5 210.82,96.52 208.28,99.06 208.28,106.68 207.01,107.95 v172.72,107.95 IC1.14 | v139.7,29.21 LED6.K
NOT_A_3  (via drill 0.8)
  Top 1.27: v170.18,105.41 170.18,81.28 147.32,58.42 147.32,35.56 146.05,34.29 144.78,34.29 142.24,31.75 138.43,31.75 135.89,29.21 v132.08,29.21
  Bottom 1.778: SV1.7 209.55,93.98 205.74,97.79 205.74,104.14 204.47,105.41 v170.18,105.41 IC1.13 | v132.08,29.21 LED5.K
NOT_A_4  (via drill 0.8)
  Top 1.27: v167.64,102.87 167.64,82.55 144.78,59.69 144.78,38.1 140.97,34.29 137.16,34.29 134.62,31.75 130.81,31.75 128.27,29.21 v124.46,29.21
  Bottom 1.778: SV1.9 208.28,91.44 203.2,96.52 203.2,101.6 201.93,102.87 v167.64,102.87 IC1.12 | v124.46,29.21 LED4.K
NOT_A_5  (via drill 0.8)
  Top 1.27: v165.1,100.33 165.1,83.82 142.24,60.96 142.24,39.37 139.7,36.83 135.89,36.83 133.35,34.29 129.54,34.29 127,31.75 123.19,31.75 120.65,29.21 v116.84,29.21
  Bottom 1.778: SV1.11 207.01,88.9 200.66,95.25 200.66,99.06 199.39,100.33 v165.1,100.33 IC1.11 | v116.84,29.21 LED3.K
NOT_A_6  (via drill 0.8)
  Top 1.27: v162.56,97.79 162.56,85.09 139.7,62.23 139.7,40.64 138.43,39.37 134.62,39.37 132.08,36.83 128.27,36.83 125.73,34.29 121.92,34.29 119.38,31.75 115.57,31.75 113.03,29.21 v109.22,29.21
  Bottom 1.778: SV1.13 205.74,86.36 198.12,93.98 198.12,96.52 196.85,97.79 v162.56,97.79 IC1.10 | v109.22,29.21 LED2.K
NOT_A_7  (via drill 0.8)
  Top 1.27: v101.6,29.21 105.41,29.21 107.95,31.75 111.76,31.75 114.3,34.29 118.11,34.29 120.65,36.83 124.46,36.83 127,39.37 130.81,39.37 133.35,41.91 135.89,41.91 137.16,43.18 137.16,63.5 160.02,86.36 v160.02,92.71
  Bottom 1.27: v160.02,92.71 184.15,92.71 193.04,83.82
  Bottom 1.778: SV1.15 193.04,83.82 IC2.16 | v101.6,29.21 LED1.K
NOT_B_0  (via drill 0.8)
  Top 1.27: v207.01,81.28 208.28,80.01 208.28,33.02 209.55,31.75 212.09,31.75 214.63,29.21 v218.44,29.21
  Bottom 1.778: SV1.19 212.09,78.74 209.55,81.28 v207.01,81.28 IC2.15 | v218.44,29.21 LED16.K
NOT_B_1  (via drill 0.8)
  Top 1.27: v205.74,78.74 205.74,30.48 207.01,29.21 v210.82,29.21
  Bottom 1.778: SV1.21 210.82,76.2 208.28,78.74 v205.74,78.74 IC2.14 | v210.82,29.21 LED15.K
NOT_B_2  (via drill 0.8)
  Top 1.27: v203.2,76.2 v203.2,29.21
  Bottom 1.778: SV1.23 209.55,73.66 207.01,76.2 v203.2,76.2 IC2.13 | v203.2,29.21 LED14.K
NOT_B_3  (via drill 0.8)
  Top 1.27: v200.66,73.66 200.66,30.48 199.39,29.21 v195.58,29.21
  Bottom 1.778: SV1.25 208.28,71.12 205.74,73.66 v200.66,73.66 IC2.12 | v195.58,29.21 LED13.K
NOT_B_4  (via drill 0.8)
  Top 1.27: v198.12,71.12 198.12,33.02 196.85,31.75 194.31,31.75 191.77,29.21 v187.96,29.21
  Bottom 1.778: SV1.27 207.01,68.58 204.47,71.12 v198.12,71.12 IC2.11 | v187.96,29.21 LED12.K
NOT_B_5  (via drill 0.8)
  Top 1.27: v195.58,68.58 195.58,35.56 194.31,34.29 193.04,34.29 190.5,31.75 186.69,31.75 184.15,29.21 v180.34,29.21
  Bottom 1.778: SV1.29 205.74,66.04 203.2,68.58 v195.58,68.58 IC2.10 | v180.34,29.21 LED11.K
NOT_B_6  (via drill 0.8)
  Top 1.27: v193.04,54.61 193.04,38.1 189.23,34.29 185.42,34.29 182.88,31.75 179.07,31.75 176.53,29.21 v172.72,29.21
  Bottom 1.778: SV1.31 210.82,63.5 209.55,62.23 209.55,55.88 208.28,54.61 v193.04,54.61 IC3.16 | v172.72,29.21 LED10.K
NOT_B_7  (via drill 0.8)
  Top 1.27: v190.5,52.07 190.5,39.37 187.96,36.83 184.15,36.83 181.61,34.29 177.8,34.29 175.26,31.75 171.45,31.75 168.91,29.21 v165.1,29.21
  Bottom 1.778: IC3.15 v190.5,52.07 210.82,52.07 213.36,54.61 SV1.33 | v165.1,29.21 LED9.K
NOT_I_0  (via drill 0.8 pad 1.78)
  Top 1.778: v222.25,73.66 222.25,57.15 v214.63,49.53
  Bottom 1.27: v214.63,49.53 219.71,49.53 243.84,25.4 LED19.K
  Bottom 1.778: SV1.24 v222.25,73.66 | IC3.14 v214.63,49.53
NOT_I_1  (via drill 0.8 pad 1.78)
  Top 1.778: v224.79,71.12 224.79,55.88 v215.9,46.99
  Bottom 1.27: v215.9,46.99 218.44,46.99 236.22,29.21 LED18.K
  Bottom 1.778: SV1.26 v224.79,71.12 | IC3.13 v215.9,46.99
NOT_I_2  (via drill 0.8 pad 1.78)
  Top 1.778: v227.33,68.58 227.33,54.61 v217.17,44.45
  Bottom 1.27: v217.17,44.45 228.6,33.02 LED17.K
  Bottom 1.778: SV1.28 v227.33,68.58 | IC3.12 v217.17,44.45
PI_A_0
  Bottom 1.27: U1.3 90.17,154.94 88.9,153.67 71.12,153.67 68.58,151.13 IC7.24
PI_A_1
  Bottom 1.27: U1.6 97.79,154.94 96.52,153.67 92.71,153.67 90.17,151.13 72.39,151.13 69.85,148.59 IC7.23
PI_A_2
  Bottom 1.27: U1.10 100.33,173.99 99.06,175.26 96.52,175.26 92.71,179.07 87.63,179.07 83.82,175.26 76.2,175.26 73.66,172.72 73.66,163.83 66.04,156.21 IC7.26
PI_A_3
  Bottom 1.27: U1.13 92.71,175.26 91.44,176.53 88.9,176.53 85.09,172.72 77.47,172.72 76.2,171.45 76.2,162.56 67.31,153.67 IC7.25
PI_A_4
  Bottom 1.27: U2.3 99.06,128.27 96.52,125.73 50.8,125.73 27.94,102.87 27.94,92.71 33.02,87.63 IC6.5
PI_A_5
  Bottom 1.27: U2.6 106.68,124.46 102.87,120.65 49.53,120.65 30.48,101.6 30.48,93.98 34.29,90.17 IC6.4
PI_A_6
  Bottom 1.27: U2.10 109.22,142.24 102.87,148.59 73.66,148.59 71.12,146.05 IC7.22
PI_A_7
  Bottom 1.27: U2.13 101.6,140.97 99.06,143.51 IC7.21
PI_B_0
  Bottom 1.27: U3.3 110.49,93.98 109.22,92.71 74.93,92.71 67.31,100.33 41.91,100.33 IC6.1
PI_B_1
  Bottom 1.27: U3.6 118.11,93.98 116.84,92.71 113.03,92.71 110.49,90.17 73.66,90.17 66.04,97.79 IC6.28
PI_B_2
  Bottom 1.27: U3.10 120.65,113.03 118.11,115.57 115.57,115.57 113.03,118.11 50.8,118.11 33.02,100.33 33.02,95.25 35.56,92.71 IC6.3
PI_B_3
  Bottom 1.27: U3.13 113.03,114.3 111.76,115.57 52.07,115.57 35.56,99.06 35.56,96.52 36.83,95.25 IC6.2
PI_B_4
  Bottom 1.27: U4.3 111.76,66.04 110.49,64.77 83.82,64.77 58.42,90.17 IC6.25
PI_B_5
  Bottom 1.27: U4.6 119.38,63.5 115.57,59.69 85.09,59.69 57.15,87.63 IC6.24
PI_B_6
  Bottom 1.27: U4.10 121.92,80.01 114.3,87.63 72.39,87.63 64.77,95.25 IC6.27
PI_B_7
  Bottom 1.27: U4.13 114.3,80.01 111.76,82.55 73.66,82.55 63.5,92.71 IC6.26
PI_I_0
  Bottom 1.27: U5.3 114.3,40.64 113.03,39.37 93.98,39.37 50.8,82.55 IC6.22
PI_I_1
  Bottom 1.27: U5.6 121.92,40.64 120.65,39.37 116.84,39.37 114.3,36.83 92.71,36.83 49.53,80.01 IC6.21
PI_I_2
  Bottom 1.27: U5.10 124.46,59.69 123.19,60.96 120.65,60.96 119.38,59.69 119.38,58.42 118.11,57.15 83.82,57.15 55.88,85.09 IC6.23
R_0
  Bottom 1.27: IC4.2 196.85,121.92 195.58,120.65 187.96,120.65 184.15,124.46 184.15,132.08 182.88,133.35 180.34,133.35 170.18,143.51 170.18,146.05 168.91,147.32 132.08,147.32 120.65,158.75 120.65,165.1 99.06,186.69 76.2,186.69 66.04,176.53 66.04,173.99 55.88,163.83 | 57.15,163.83 55.88,163.83 | 55.88,163.83 IC7.1
R_1
  Bottom 1.27: IC4.4 201.93,119.38 200.66,118.11 186.69,118.11 181.61,123.19 181.61,129.54 180.34,130.81 179.07,130.81 167.64,142.24 167.64,143.51 166.37,144.78 130.81,144.78 118.11,157.48 118.11,163.83 97.79,184.15 77.47,184.15 68.58,175.26 68.58,166.37 63.5,161.29 IC7.28
R_2
  Bottom 1.27: IC4.6 207.01,119.38 203.2,115.57 185.42,115.57 179.07,121.92 179.07,127 163.83,142.24 129.54,142.24 115.57,156.21 115.57,162.56 96.52,181.61 78.74,181.61 71.12,173.99 71.12,165.1 64.77,158.75 IC7.27
R_3
  Bottom 1.27: IC4.10 209.55,137.16 205.74,140.97 184.15,140.97 177.8,147.32 177.8,153.67 176.53,154.94 135.89,154.94 128.27,162.56 128.27,168.91 102.87,194.31 72.39,194.31 44.45,166.37 44.45,157.48 48.26,153.67 IC7.4
R_4
  Bottom 1.27: IC4.12 204.47,134.62 200.66,138.43 182.88,138.43 175.26,146.05 175.26,151.13 173.99,152.4 134.62,152.4 125.73,161.29 125.73,167.64 101.6,191.77 73.66,191.77 46.99,165.1 46.99,158.75 49.53,156.21 IC7.3
R_5
  Bottom 1.27: IC4.15 196.85,134.62 195.58,135.89 181.61,135.89 172.72,144.78 172.72,148.59 171.45,149.86 133.35,149.86 123.19,160.02 123.19,166.37 100.33,189.23 74.93,189.23 49.53,163.83 49.53,160.02 50.8,158.75 IC7.2
R_6
  Bottom 1.27: IC5.2 196.85,149.86 195.58,148.59 187.96,148.59 185.42,151.13 185.42,161.29 184.15,162.56 139.7,162.56 135.89,166.37 135.89,172.72 106.68,201.93 68.58,201.93 36.83,170.18 36.83,153.67 44.45,146.05 IC7.7
R_7
  Bottom 1.27: IC5.4 201.93,147.32 200.66,146.05 186.69,146.05 182.88,149.86 182.88,158.75 181.61,160.02 138.43,160.02 133.35,165.1 133.35,171.45 105.41,199.39 69.85,199.39 39.37,168.91 39.37,154.94 45.72,148.59 IC7.6
R_8
  Bottom 1.27: IC5.6 207.01,147.32 203.2,143.51 185.42,143.51 180.34,148.59 180.34,156.21 179.07,157.48 137.16,157.48 130.81,163.83 130.81,170.18 104.14,196.85 71.12,196.85 41.91,167.64 41.91,156.21 46.99,151.13 IC7.5
RESULT_0  (via drill 0.8 pad 1.78)
  Top 1.778: v199.39,120.65 204.47,115.57 v215.9,115.57
  Bottom 1.778: R28.2 215.9,180.34 v215.9,115.57 SV1.2 | IC4.3 v199.39,120.65
RESULT_1  (via drill 0.8 pad 1.78)
  Top 1.778: v204.47,120.65 207.01,118.11 v218.44,118.11
  Bottom 1.778: SV1.4 217.17,99.06 218.44,100.33 v218.44,118.11 218.44,181.61 213.36,186.69 205.74,186.69 R27.2 | IC4.5 v204.47,120.65
RESULT_2  (via drill 0.8 pad 1.78)
  Top 1.778: v209.55,120.65 v220.98,120.65
  Bottom 1.778: SV1.6 218.44,96.52 220.98,99.06 v220.98,120.65 220.98,182.88 214.63,189.23 199.39,189.23 R26.2 | IC4.7 v209.55,120.65
RESULT_3  (via drill 0.8 pad 1.78)
  Top 1.778: v212.09,135.89 v223.52,135.89
  Bottom 1.778: SV1.8 219.71,93.98 223.52,97.79 v223.52,135.89 223.52,184.15 215.9,191.77 193.04,191.77 R25.2 | v212.09,135.89 IC4.9
RESULT_4  (via drill 0.8 pad 1.78)
  Top 1.778: v207.01,135.89 209.55,138.43 v226.06,138.43
  Bottom 1.778: SV1.10 220.98,91.44 226.06,96.52 v226.06,138.43 226.06,185.42 217.17,194.31 186.69,194.31 R24.2 | v207.01,135.89 IC4.11
RESULT_5  (via drill 0.8 pad 1.78)
  Top 1.778: v199.39,135.89 204.47,140.97 v228.6,140.97
  Bottom 1.778: SV1.12 222.25,88.9 228.6,95.25 v228.6,140.97 228.6,186.69 218.44,196.85 180.34,196.85 R23.2 | v199.39,135.89 IC4.14
RESULT_6  (via drill 0.8)
  Top 1.778: v199.39,148.59 204.47,143.51 v231.14,143.51
  Bottom 1.778: SV1.14 223.52,86.36 231.14,93.98 v231.14,143.51 231.14,187.96 219.71,199.39 173.99,199.39 R22.2 | IC5.3 v199.39,148.59
RESULT_7  (via drill 0.8)
  Top 1.778: v204.47,148.59 207.01,146.05 v233.68,146.05
  Bottom 1.778: SV1.16 224.79,83.82 233.68,92.71 v233.68,146.05 233.68,189.23 220.98,201.93 167.64,201.93 R21.2 | IC5.5 v204.47,148.59
SELECT  (via drill 0.8)
  Top 1.27: v59.69,77.47 59.69,85.09 v63.5,88.9 63.5,99.06 v67.31,102.87 v67.31,130.81 67.31,148.59 v74.93,156.21 74.93,157.48 48.26,184.15 48.26,194.31 C9.1 R33.2 R53.2
  Bottom 1.27: 104.14,69.85 U4.1 82.55,69.85 v63.5,88.9 | U2.1 v67.31,130.81 | U5.1 90.17,46.99 v59.69,77.47 | U3.1 71.12,100.33 68.58,102.87 v67.31,102.87 | U1.1 80.01,156.21 v74.93,156.21
  Bottom 1.778: C9.1 R33.2 R53.2
SW_A_0  (via drill 0.8)
  Top 1.27: R34.2 41.91,24.13 41.91,33.02 43.18,34.29 44.45,34.29 46.99,36.83 48.26,36.83 50.8,39.37 52.07,39.37 54.61,41.91 55.88,41.91 58.42,44.45 59.69,44.45 62.23,46.99 63.5,46.99 66.04,49.53 67.31,49.53 69.85,52.07 71.12,52.07 73.66,54.61 74.93,54.61 78.74,58.42 78.74,66.04 81.28,68.58 81.28,71.12 83.82,73.66 83.82,81.28 86.36,83.82 86.36,86.36 87.63,87.63 87.63,129.54 85.09,132.08 85.09,139.7 87.63,142.24 v87.63,156.21
  Bottom 1.27: SW1.1 R34.2 | U1.2 v87.63,156.21
SW_A_1  (via drill 0.8)
  Top 1.27: R35.2 36.83,24.13 36.83,33.02 38.1,34.29 39.37,34.29 41.91,36.83 43.18,36.83 45.72,39.37 46.99,39.37 49.53,41.91 50.8,41.91 53.34,44.45 54.61,44.45 57.15,46.99 58.42,46.99 60.96,49.53 62.23,49.53 64.77,52.07 66.04,52.07 68.58,54.61 69.85,54.61 72.39,57.15 73.66,57.15 76.2,59.69 76.2,67.31 78.74,69.85 78.74,72.39 81.28,74.93 81.28,82.55 83.82,85.09 83.82,87.63 85.09,88.9 85.09,128.27 82.55,130.81 82.55,140.97 85.09,143.51 85.09,157.48 86.36,158.75 88.9,158.75 90.17,157.48 90.17,156.21 91.44,154.94 93.98,154.94 v95.25,156.21
  Bottom 1.27: SW1.2 27.94,15.24 R35.2 | U1.5 v95.25,156.21
SW_A_2  (via drill 0.8)
  Top 1.27: R36.2 31.75,24.13 31.75,33.02 33.02,34.29 34.29,34.29 36.83,36.83 38.1,36.83 40.64,39.37 41.91,39.37 44.45,41.91 45.72,41.91 48.26,44.45 49.53,44.45 52.07,46.99 53.34,46.99 55.88,49.53 57.15,49.53 59.69,52.07 60.96,52.07 63.5,54.61 64.77,54.61 67.31,57.15 68.58,57.15 71.12,59.69 72.39,59.69 73.66,60.96 73.66,68.58 76.2,71.12 76.2,73.66 78.74,76.2 78.74,83.82 81.28,86.36 81.28,88.9 82.55,90.17 82.55,127 80.01,129.54 80.01,142.24 82.55,144.78 82.55,160.02 81.28,161.29 78.74,161.29 77.47,162.56 77.47,170.18 78.74,171.45 96.52,171.45 v97.79,172.72
  Bottom 1.27: SW1.3 25.4,17.78 R36.2 | U1.11 v97.79,172.72
SW_A_3  (via drill 0.8)
  Top 1.27: R37.2 26.67,24.13 26.67,33.02 27.94,34.29 29.21,34.29 31.75,36.83 33.02,36.83 35.56,39.37 36.83,39.37 39.37,41.91 40.64,41.91 43.18,44.45 44.45,44.45 46.99,46.99 48.26,46.99 50.8,49.53 52.07,49.53 54.61,52.07 55.88,52.07 58.42,54.61 59.69,54.61 62.23,57.15 63.5,57.15 66.04,59.69 67.31,59.69 71.12,63.5 71.12,69.85 73.66,72.39 73.66,74.93 76.2,77.47 76.2,85.09 78.74,87.63 78.74,90.17 80.01,91.44 80.01,125.73 77.47,128.27 77.47,143.51 80.01,146.05 80.01,157.48 78.74,158.75 77.47,158.75 74.93,161.29 74.93,171.45 77.47,173.99 v90.17,173.99
  Bottom 1.27: SW1.4 22.86,20.32 R37.2 | U1.14 v90.17,173.99
SW_A_4  (via drill 0.8)
  Top 1.27: R38.2 21.59,24.13 21.59,33.02 22.86,34.29 24.13,34.29 26.67,36.83 27.94,36.83 30.48,39.37 31.75,39.37 34.29,41.91 35.56,41.91 38.1,44.45 39.37,44.45 41.91,46.99 43.18,46.99 45.72,49.53 46.99,49.53 49.53,52.07 50.8,52.07 53.34,54.61 54.61,54.61 57.15,57.15 58.42,57.15 60.96,59.69 62.23,59.69 64.77,62.23 66.04,62.23 68.58,64.77 68.58,71.12 71.12,73.66 71.12,76.2 73.66,78.74 73.66,86.36 76.2,88.9 76.2,91.44 77.47,92.71 77.47,124.46 74.93,127 v74.93,128.27
  Bottom 1.27: SW1.5 20.32,20.32 R38.2 | U2.2 96.52,129.54 95.25,128.27 v74.93,128.27
SW_A_5  (via drill 0.8)
  Top 1.27: R39.2 16.51,24.13 16.51,33.02 17.78,34.29 19.05,34.29 21.59,36.83 22.86,36.83 25.4,39.37 26.67,39.37 29.21,41.91 30.48,41.91 33.02,44.45 34.29,44.45 36.83,46.99 38.1,46.99 40.64,49.53 41.91,49.53 44.45,52.07 45.72,52.07 48.26,54.61 49.53,54.61 52.07,57.15 53.34,57.15 55.88,59.69 57.15,59.69 59.69,62.23 60.96,62.23 63.5,64.77 64.77,64.77 66.04,66.04 66.04,72.39 68.58,74.93 68.58,77.47 71.12,80.01 71.12,87.63 73.66,90.17 73.66,92.71 74.93,93.98 v74.93,123.19
  Bottom 1.27: SW1.6 17.78,17.78 R39.2 | U2.5 104.14,125.73 101.6,123.19 v74.93,123.19
SW_A_6  (via drill 0.8)
  Top 1.27: R40.2 11.43,24.13 11.43,33.02 12.7,34.29 13.97,34.29 16.51,36.83 17.78,36.83 20.32,39.37 21.59,39.37 24.13,41.91 25.4,41.91 27.94,44.45 29.21,44.45 31.75,46.99 33.02,46.99 35.56,49.53 36.83,49.53 39.37,52.07 40.64,52.07 43.18,54.61 44.45,54.61 46.99,57.15 48.26,57.15 50.8,59.69 52.07,59.69 54.61,62.23 55.88,62.23 58.42,64.77 59.69,64.77 63.5,68.58 63.5,73.66 66.04,76.2 66.04,78.74 68.58,81.28 68.58,88.9 71.12,91.44 71.12,93.98 72.39,95.25 72.39,129.54 74.93,132.08 v74.93,146.05
  Bottom 1.27: SW1.7 15.24,15.24 R40.2 | U2.11 106.68,139.7 100.33,146.05 v74.93,146.05
SW_A_7  (via drill 0.8)
  Top 1.27: R41.2 6.35,24.13 6.35,33.02 7.62,34.29 8.89,34.29 11.43,36.83 12.7,36.83 15.24,39.37 16.51,39.37 19.05,41.91 20.32,41.91 22.86,44.45 24.13,44.45 26.67,46.99 27.94,46.99 30.48,49.53 31.75,49.53 34.29,52.07 35.56,52.07 38.1,54.61 39.37,54.61 41.91,57.15 43.18,57.15 45.72,59.69 46.99,59.69 49.53,62.23 50.8,62.23 53.34,64.77 54.61,64.77 57.15,67.31 58.42,67.31 60.96,69.85 60.96,74.93 63.5,77.47 63.5,80.01 66.04,82.55 66.04,90.17 68.58,92.71 68.58,95.25 69.85,96.52 69.85,130.81 72.39,133.35 v72.39,140.97
  Bottom 1.27: SW1.8 R41.2 | U2.14 99.06,139.7 97.79,140.97 v72.39,140.97
SW_B_0  (via drill 0.8)
  Top 1.27: R42.2 82.55,24.13 82.55,33.02 83.82,34.29 85.09,34.29 87.63,36.83 88.9,36.83 99.06,46.99 99.06,86.36 v107.95,95.25
  Bottom 1.27: SW2.1 R42.2 | U3.2 v107.95,95.25
SW_B_1  (via drill 0.8)
  Top 1.27: R43.2 77.47,24.13 77.47,33.02 78.74,34.29 80.01,34.29 82.55,36.83 83.82,36.83 86.36,39.37 87.63,39.37 96.52,48.26 96.52,87.63 106.68,97.79 109.22,97.79 110.49,96.52 110.49,95.25 111.76,93.98 114.3,93.98 v115.57,95.25
  Bottom 1.27: SW2.2 68.58,15.24 R43.2 | U3.5 v115.57,95.25
SW_B_2  (via drill 0.8)
  Top 1.27: R44.2 72.39,24.13 72.39,33.02 73.66,34.29 74.93,34.29 77.47,36.83 78.74,36.83 81.28,39.37 82.55,39.37 85.09,41.91 86.36,41.91 93.98,49.53 93.98,88.9 97.79,92.71 97.79,109.22 99.06,110.49 116.84,110.49 v118.11,111.76
  Bottom 1.27: SW2.3 66.04,17.78 R44.2 | U3.11 v118.11,111.76
SW_B_3  (via drill 0.8)
  Top 1.27: R45.2 67.31,24.13 67.31,33.02 68.58,34.29 69.85,34.29 72.39,36.83 73.66,36.83 76.2,39.37 77.47,39.37 80.01,41.91 81.28,41.91 83.82,44.45 85.09,44.45 91.44,50.8 91.44,90.17 95.25,93.98 95.25,111.76 96.52,113.03 v110.49,113.03
  Bottom 1.27: R45.2 63.5,20.32 SW2.4 | U3.14 v110.49,113.03
SW_B_4  (via drill 0.8)
  Top 1.27: R46.2 62.23,24.13 62.23,33.02 63.5,34.29 64.77,34.29 67.31,36.83 68.58,36.83 71.12,39.37 72.39,39.37 74.93,41.91 76.2,41.91 78.74,44.45 80.01,44.45 82.55,46.99 83.82,46.99 88.9,52.07 v88.9,67.31
  Bottom 1.27: R46.2 60.96,20.32 SW2.5 | U4.2 109.22,68.58 107.95,67.31 v88.9,67.31
SW_B_5  (via drill 0.8)
  Top 1.27: R47.2 57.15,24.13 57.15,33.02 58.42,34.29 59.69,34.29 62.23,36.83 63.5,36.83 66.04,39.37 67.31,39.37 69.85,41.91 71.12,41.91 73.66,44.45 74.93,44.45 77.47,46.99 78.74,46.99 86.36,54.61 v86.36,62.23
  Bottom 1.27: SW2.6 58.42,17.78 R47.2 | U4.5 116.84,64.77 114.3,62.23 v86.36,62.23
SW_B_6  (via drill 0.8)
  Top 1.27: R48.2 52.07,24.13 52.07,33.02 53.34,34.29 54.61,34.29 57.15,36.83 58.42,36.83 60.96,39.37 62.23,39.37 64.77,41.91 66.04,41.91 68.58,44.45 69.85,44.45 72.39,46.99 73.66,46.99 76.2,49.53 77.47,49.53 83.82,55.88 83.82,63.5 86.36,66.04 86.36,68.58 88.9,71.12 v88.9,85.09
  Bottom 1.27: SW2.7 55.88,15.24 R48.2 | U4.11 119.38,78.74 113.03,85.09 v88.9,85.09
SW_B_7  (via drill 0.8)
  Top 1.27: R49.2 46.99,24.13 46.99,33.02 48.26,34.29 49.53,34.29 52.07,36.83 53.34,36.83 55.88,39.37 57.15,39.37 59.69,41.91 60.96,41.91 63.5,44.45 64.77,44.45 67.31,46.99 68.58,46.99 71.12,49.53 72.39,49.53 74.93,52.07 76.2,52.07 81.28,57.15 81.28,64.77 83.82,67.31 83.82,69.85 86.36,72.39 v86.36,80.01
  Bottom 1.27: SW2.8 R49.2 | U4.14 111.76,78.74 110.49,80.01 v86.36,80.01
SW_I_0  (via drill 0.8)
  Top 1.27: v111.76,41.91 111.76,35.56 110.49,34.29 106.68,34.29 104.14,31.75 100.33,31.75 97.79,29.21 97.79,24.13 R50.2
  Bottom 1.27: SW3.1 92.71,19.05 R50.2 | U5.2 v111.76,41.91
SW_I_1  (via drill 0.8)
  Top 1.27: R51.2 92.71,24.13 92.71,33.02 93.98,34.29 102.87,34.29 105.41,36.83 107.95,36.83 109.22,38.1 109.22,43.18 110.49,44.45 113.03,44.45 114.3,43.18 114.3,41.91 115.57,40.64 118.11,40.64 v119.38,41.91
  Bottom 1.27: SW3.2 R51.2 | U5.5 v119.38,41.91
SW_I_2  (via drill 0.8)
  Top 1.27: R52.2 87.63,24.13 87.63,33.02 88.9,34.29 90.17,34.29 101.6,45.72 101.6,55.88 102.87,57.15 120.65,57.15 v121.92,58.42
  Bottom 1.27: SW3.3 87.63,19.05 R52.2 | U5.11 v121.92,58.42

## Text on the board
Top: Control Board / Topside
